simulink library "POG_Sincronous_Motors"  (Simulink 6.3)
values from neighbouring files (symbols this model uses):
  al = Tipo(2)    [Flusso_Rotorico_An.m]
  bm = 0.8*N*metri*secondo/rad    (= 0.8)    [architetture_epicicloidale.m]    (also in architetture_epicicloidale_cont.m; architetture_epicicloidale_HEV.m; architetture_epicicloidale_prova.m; architetture_HEV_controllo.m)
  Iw0 = 0*wI0    [architetture_epicicloidale.m]    (also in architetture_epicicloidale_cont.m = wI0; architetture_epicicloidale_HEV.m; architetture_epicicloidale_prova.m; architetture_HEV_controllo.m)
  Jm = 1.6*kg*metri^2    (= 1.6)    [architetture_epicicloidale.m]    (also in architetture_epicicloidale_cont.m; architetture_epicicloidale_HEV.m = 1.64945909552; architetture_epicicloidale_prova.m; architetture_HEV_controllo.m = 0.529459095518)
  m = 5    [architetture_epicicloidale.m]    (also in architetture_epicicloidale_cont.m; architetture_epicicloidale_HEV.m; architetture_epicicloidale_prova.m; architetture_HEV_controllo.m)
  Nar = 200    [architetture_epicicloidale.m]    (also in architetture_epicicloidale_cont.m; architetture_epicicloidale_HEV.m; architetture_epicicloidale_prova.m; architetture_HEV_controllo.m)
  Nc = 30    [architetture_epicicloidale.m]    (also in architetture_epicicloidale_cont.m; architetture_epicicloidale_HEV.m; architetture_epicicloidale_prova.m; architetture_HEV_controllo.m)
  p = 1    [architetture_epicicloidale.m]    (also in architetture_epicicloidale_cont.m; architetture_epicicloidale_HEV.m; architetture_epicicloidale_prova.m; architetture_HEV_controllo.m)
  Phir = 0.02*Weber    (= 0.02)    [architetture_epicicloidale.m]    (also in architetture_epicicloidale_cont.m; architetture_epicicloidale_HEV.m; architetture_epicicloidale_prova.m; architetture_HEV_controllo.m)
  Star = Si    [architetture_epicicloidale.m]    (also in architetture_epicicloidale_cont.m; architetture_epicicloidale_HEV.m; architetture_epicicloidale_prova.m; architetture_HEV_controllo.m)
  Thm0 = 0    [architetture_epicicloidale.m]    (also in architetture_epicicloidale_cont.m; architetture_epicicloidale_HEV.m; architetture_epicicloidale_prova.m; architetture_HEV_controllo.m)
  Tipo = eval(Flusso(ij).Tipo)    [architetture_epicicloidale.m]    (also in architetture_epicicloidale_cont.m; architetture_epicicloidale_HEV.m; architetture_epicicloidale_prova.m; architetture_HEV_controllo.m)
  Wm0 = 0*Wr_d    (= 0)    [architetture_epicicloidale.m]    (also in architetture_epicicloidale_cont.m = 62.5; architetture_epicicloidale_HEV.m; architetture_epicicloidale_prova.m; architetture_HEV_controllo.m)
undefined symbols (not defined in the file or in its folder): Ls, Ms0, Rs
libraries: simulink x2

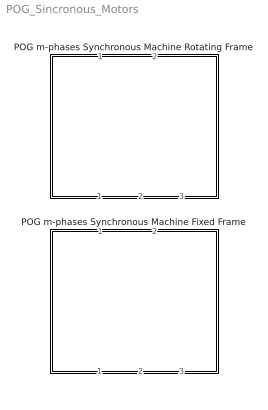
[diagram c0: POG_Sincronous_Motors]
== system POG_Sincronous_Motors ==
  POG m-phases Synchronous Machine Fixed Frame : Subsystem  Orientation=down  mask(POG Multi-Phase Motor (Fixed Frame)){Motor_Par=[m p], Phase_Par=[Nc Star], Electric_Par=[Rs Ls Ms0], Mech_Par=[Jm bm], Plux_Par=[Phir Nar], Iniz_Cond=[Wm0; Thm0; Iw0], TipoFlux=User defined, Tipo=Tipo, alfa=al, degree=6, TipoF=Tipo}
      mask prompts: Motor_Par "Number of phases, Number of polar couples: [m, p] -> [Nr, Nr]"; Phase_Par "Number of coils, Star connected?: [Nc, Star] -> [Nr, (True, False)]"; Electric_Par "Electric Parameters: [Rs, Ls, Ms0] -> [Henry, Henry, Ohm]"; Mech_Par "Mechanical Parameters: [Jm, bm] -> [kg*m^2, N m s/rad]"; Plux_Par "Maximum value of the rotor flux, Number of Fourier harmonics: [Phir, Nar] -> [W, Nr]"; Iniz_Cond "Initial conditions: [Wm0, Thm0, It0] -> [rad/s, rad, A]"; TipoFlux "Type of Rotor Flux"; Tipo "Type defined by user: Tipo -> [Nr,alfa,degree]"; alfa "Flux function parameter: alfa -> [0, pi/2]:"; degree "Degree of the polinomial flux function:"; TipoF "Components of the Fourier series: [9, Nmax, CompAi] -> [9, Nr, a0, a1, ..., aNr]"
      mask help: Multi-Phase Permanent Magnet Synchronous Motor: [m, p] = Number of motor phases, Polar couples; [Nc, Star] = Number of coils per phase, Type of phase connection; [Rs, Ls, Ms0] = Resistance, Self inductance, Mutual inductance of each phase; [Jm, bm] = Inertia momentum, Friction coefficient of the rotor; [Phir, Nar] = Maximum value of the rotor flux, Number of Fourier harmonics; [Wm0, Thm0, Iw0] = Initial conditions on Velocity, Position of the motor and Currents; Type of Rotor Flux (Tipo): Trapezoidal [1,alfa]; Triangular [1, 0]; Squared wave [2]; Sinusoidal [3]; Cosinusoidally connected [4,alf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
      mask init:
      | m=Motor_Par(1);
      | p=Motor_Par(2);
      | Nc=Phase_Par(1);
      | Star=Phase_Par(2);
      | Rs=Electric_Par(1);
      | Ls=Electric_Par(2);
      | Ms0=Electric_Par(3);
      | Jm=Mech_Par(1);
      | bm=Mech_Par(2);
      | Phir=Plux_Par(1);
      | Nar=Plux_Par(2);
      | 
      | %%%%%%%%%%%%%%%%%%%%% Initial Conditions
      | if length(Iniz_Cond)<(m+2-Star)
      |     Iniz_Cond=[Iniz_Cond 0*[1:m+2-Star-length(Iniz_Cond)]];
      |     disp('Correction: Iniz_Cond = ...');
      |     disp(Iniz_Cond)
      | end
      | Wm0 = Iniz_Cond(1);
      | Thm0= Iniz_Cond(2);
      | Ibt0 = Iniz_Cond(3:m+2-Star);
      | 
      | %%%%%%%%%%%%%%%%%%%%%%%%%%%%
      | FluxName(1)=struct('Nome','Trapezoidal');
      | FluxName(2)=struct('Nome','Squared wave');
      | FluxName(3)=struct('Nome','Sinusoidal');
      | FluxName(4)=struct('Nome','Cosinusoidally connected');
      | FluxName(5)=struct('Nome','Sinusoidally connected');
      | FluxName(6)=struct('Nome','Polynomial even');
      | FluxName(7)=struct('Nome','Polynomial odd');
      | FluxName(8)=struct('Nome','Trapezoidal if derived');
      | FluxName(9)=struct('Nome','Fourier defined');
      | 
      | switch TipoFlux
      |     case 'User defined',
      |     case 'Trapezoidal'
      |         if alfa<0, alfa=0; disp('Correction: alfa = 0'); end
      |         if alfa>pi/2, alfa=pi/2; disp('Correction: alfa = pi/2'); end
      |         Tipo = [1,alfa];
      |     case 'Triangular'
      |         Tipo = [1,  0];
      |     case 'Squared wave'
      |         Tipo = [2];
      |     case 'Sinusoidal'
      |         Tipo = [3];
      |     case 'Cosinusoidally connected'
      |         if alfa<0, alfa=0; disp('Correction: alfa = 0'); end
      |         if alfa>pi/2, alfa=pi/2; disp('Correction: alfa = pi/2'); end
      |         Tipo = [4,alfa];
      |     case 'Sinusoidally connected'
      |         if alfa<0, alfa=0; disp('Correction: alfa = 0'); end
      |         if alfa>pi/2, alfa=pi/2; disp('Correction: alfa = pi/2'); end
      |         Tipo = [5,alfa];
      |     case 'Polynomial even'
      |         if alfa<0, alfa=0; disp('Correction: alfa = 0'); end
      |         if alfa>pi/2, alfa=pi/2; disp('Correction: alfa = pi/2'); end
      |         if rem(degree)==1, 
      |             degree=degree-1; 
      |             disp(['Correction: degree = ' num2str(degree)]); 
      |         end
      |         if degree<2
      |             degree=2; 
      |             disp(['Correction: degree = ' num2str(degree)]); 
      |         end            
      |         Tipo = [6,alfa,degree];
      |     case 'Polynomial odd'
      |         if alfa<0, alfa=0; disp('Correction: alfa = 0'); end
      |         if alfa>pi/2, alfa=pi/2; disp('Correction: alfa = pi/2'); end
      |         if rem(degree)==0, 
      |             degree=degree-1; 
      |             disp(['Correction: degree = ' num2str(degree)]); 
      |         end
      |         if degree<1
      |             degree=1; 
      |             disp(['Correction: degree = ' num2str(degree)]); 
      |         end            
      |         Tipo = [7,alfa,degree];
      |     case 'Trapezoidal if derived'
      |         Tipo = [8,alfa];
      |         if alfa<0, alfa=0; disp('Correction: alfa = 0'); end
      |         if alfa>pi/2, alfa=pi/2; disp('Correction: alfa = pi/2'); end
      |     case 'Fourier defined'
      |         if TipoF(1)~=9
      |             disp('Correction: NrType = 9 (Fourier defined)')
      |             TipoF(1)=9;
      |         end
      |         if length(TipoF)<2
      |             TipoF(2)=m;
      |             disp('Correction: Fourier defined -> TipoF = ...');
      |             disp(TipoF)
      |         end
      |         if TipoF(2)<m,
      |             TipoF(2)=m;
      |             disp('Correction: Fourier defined -> Nas = m');
      |         end
      |         if length(TipoF)<(TipoF(2)+3)
      |             TipoF=[TipoF 0*[1:TipoF(2)+3-length(TipoF)]];
      |             disp('Correction: Fourier defined -> TipoF = ...'); 
      |             disp(TipoF)
      |         end
      |         Tipo = TipoF;   % [9,Nmax,CompAi]
      |     otherwise,
      |         disp('Flux type not correct')
      |         return
      | end
      | 
      | switch TipoFlux
      |     case 'User defined',
      |         disp(['The rotor flux is ''''' FluxName(Tipo(1)).Nome ''''' (Us. Def.)'])
      |     otherwise,
      |         disp(['The rotor flux is ''''' TipoFlux ''''''])
      | end
      | 
      | %%%%%% Trasformazione "T(b->t)"
      | %%%%%% matrice tTb=T_b_Concordia_Sincrono(m); 
      | if rem(m,2)==0
      |     disp(['Warning (T_b_Concordia_Sincrono): m = ' num2str(m) ' è pari']) 
      | end
      | tTb = ones(m)/sqrt(2);
      | w = 2*pi/m;
      | for k = [1:2:m-2]
      |     for h = [0:m-1]
      |         tTb(h+1,k  ) = cos(h*k*w);
      |         tTb(h+1,k+1) = sin(h*k*w);
      |     end
      | end
      | tTb=sqrt(2/m)*tTb;
      | 
      | %%%%%% Auto and mutual inductance matrix  wLs(MLb) defined in the rotating frame
      | Ls0 = Ls-Ms0;
      | MLb = p*eye(m)*Ls0;         
      | MLb(1,1)=p*(Ls0+m*Ms0/2);  
      | MLb(2,2)=p*(Ls0+m*Ms0/2);
      | 
      | %%%%%% Resistance matrice wRs(MR) defined in the rotating frame
      | MR = p*Rs*eye(m);   
      | 
      | %%%%%% Calcolo del vetore di coppia Ktau
      | Phic = p*Nc*Phir;   %%% Maximum concatenated flux;
      | if Nar<m,           %%% Nar = numero di compenenti spettrali dello svilupo in serie
      |     Nar=m;  disp('Correction: Nar = m');
      | end
      | 
      | %%%%%% Reduction of the system matrices if Star is True
      | if Star                     
      |     tTabc=tTb(:,[1:m-1]);
      |     MLabc=MLb([1:m-1],[1:m-1]);
      |     MRabc=MR([1:m-1],[1:m-1]);
      |     Ibt0=MLabc*Ibt0;
      | else
      |     tTabc=eye(m);
      |     MLabc=tTb*MLb*tTb';
      |     MRabc=tTb*MR*tTb';
      |     Ibt0=MLabc*tTabc'*Ibt0;
      | end
      | Sfasa  = -2*pi*[0:m-1]'/m;   % Matrice di sfasamento
      | LkUpT_in=[-1:0.0001:1]*2*pi;
      | LkUpT_out=0*LkUpT_in;
      | for n=[1:2:Nar]
      |     LkUpT_out=LkUpT_out-Flusso_Rotorico_An(Tipo,n)*n*sin(n*LkUpT_in);
      | end
      | LkUpT_out=p*Phic*LkUpT_out;
  POG m-phases Synchronous Machine Rotating Frame : Subsystem  Orientation=down  mask(POG Multi-Phase Motor (Rotating Frame)){Motor_Par=[m p], Phase_Par=[Nc Star], Electric_Par=[Rs Ls Ms0], Mech_Par=[Jm bm], Plux_Par=[Phir Nar], Iniz_Cond=[Wm0; Thm0; Iw0], TipoFlux=User defined, Tipo=Tipo, alfa=al, degree=6, TipoF=Tipo}
      mask prompts: Motor_Par "Number of phases, Number of polar couples: [m, p] -> [Nr, Nr]"; Phase_Par "Number of coils, Star connected?: [Nc, Star] -> [Nr, (True, False)]"; Electric_Par "Electric Parameters: [Rs, Ls, Ms0] -> [Henry, Henry, Ohm]"; Mech_Par "Mechanical Parameters: [Jm, bm] -> [kg*m^2, N m s/rad]"; Plux_Par "Maximum value of the rotor flux, Number of Fourier harmonics: [Phir, Nar] -> [W, Nr]"; Iniz_Cond "Initial conditions: [Wm0, Thm0, Iw0] -> [rad/s, rad, A]"; TipoFlux "Type of Rotor Flux"; Tipo "Type defined by user: Tipo -> [Nr,alfa,degree]"; alfa "Flux function parameter: alfa -> [0, pi/2]:"; degree "Degree of the polinomial flux function:"; TipoF "Components of the Fourier series: [9, Nmax, CompAi] -> [9, Nr, a0, a1, ..., aNr]"
      mask help: Multi-Phase Permanent Magnet Synchronous Motor: [m, p] = Number of motor phases, Polar couples; [Nc, Star] = Number of coils per phase, Type of phase connection; [Rs, Ls, Ms0] = Resistance, Self inductance, Mutual inductance of each phase; [Jm, bm] = Inertia momentum, Friction coefficient of the rotor; [Phir, Nar] = Maximum value of the rotor flux, Number of Fourier harmonics; [Wm0, Thm0, Iw0] = Initial conditions on Velocity, Position of the motor and Currents; Type of Rotor Flux (Tipo): Trapezoidal [1,alfa]; Triangular [1, 0]; Squared wave [2]; Sinusoidal [3]; Cosinusoidally connected [4,alf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
      mask init:
      | m=Motor_Par(1);
      | p=Motor_Par(2);
      | Nc=Phase_Par(1);
      | Star=Phase_Par(2);
      | Rs=Electric_Par(1);
      | Ls=Electric_Par(2);
      | Ms0=Electric_Par(3);
      | Jm=Mech_Par(1);
      | bm=Mech_Par(2);
      | Phir=Plux_Par(1);
      | Nar=Plux_Par(2);
      | 
      | %%%%%%%%%%%%%%%%%%%%% Initial Conditions
      | if length(Iniz_Cond)<(m+2-Star)
      |     Iniz_Cond=[Iniz_Cond 0*[1:m+2-Star-length(Iniz_Cond)]];
      |     disp('Correction: Iniz_Cond = ...');
      |     disp(Iniz_Cond)
      | end
      | Wm0 = Iniz_Cond(1);
      | Thm0= Iniz_Cond(2);
      | Iw0 = Iniz_Cond(3:m+2-Star);
      | 
      | %%%%%%%%%%%%%%%%%%%%%%%%%%%%
      | FluxName(1)=struct('Nome','Trapezoidal');
      | FluxName(2)=struct('Nome','Squared wave');
      | FluxName(3)=struct('Nome','Sinusoidal');
      | FluxName(4)=struct('Nome','Cosinusoidally connected');
      | FluxName(5)=struct('Nome','Sinusoidally connected');
      | FluxName(6)=struct('Nome','Polynomial even');
      | FluxName(7)=struct('Nome','Polynomial odd');
      | FluxName(8)=struct('Nome','Trapezoidal if derived');
      | FluxName(9)=struct('Nome','Fourier defined');
      | 
      | switch TipoFlux
      |     case 'User defined',
      |     case 'Trapezoidal'
      |         if alfa<0, alfa=0; disp('Correction: alfa = 0'); end
      |         if alfa>pi/2, alfa=pi/2; disp('Correction: alfa = pi/2'); end
      |         Tipo = [1,alfa];
      |     case 'Triangular'
      |         Tipo = [1,  0];
      |     case 'Squared wave'
      |         Tipo = [2];
      |     case 'Sinusoidal'
      |         Tipo = [3];
      |     case 'Cosinusoidally connected'
      |         if alfa<0, alfa=0; disp('Correction: alfa = 0'); end
      |         if alfa>pi/2, alfa=pi/2; disp('Correction: alfa = pi/2'); end
      |         Tipo = [4,alfa];
      |     case 'Sinusoidally connected'
      |         if alfa<0, alfa=0; disp('Correction: alfa = 0'); end
      |         if alfa>pi/2, alfa=pi/2; disp('Correction: alfa = pi/2'); end
      |         Tipo = [5,alfa];
      |     case 'Polynomial even'
      |         if alfa<0, alfa=0; disp('Correction: alfa = 0'); end
      |         if alfa>pi/2, alfa=pi/2; disp('Correction: alfa = pi/2'); end
      |         if rem(degree)==1, 
      |             degree=degree-1; 
      |             disp(['Correction: degree = ' num2str(degree)]); 
      |         end
      |         if degree<2
      |             degree=2; 
      |             disp(['Correction: degree = ' num2str(degree)]); 
      |         end            
      |         Tipo = [6,alfa,degree];
      |     case 'Polynomial odd'
      |         if alfa<0, alfa=0; disp('Correction: alfa = 0'); end
      |         if alfa>pi/2, alfa=pi/2; disp('Correction: alfa = pi/2'); end
      |         if rem(degree)==0, 
      |             degree=degree-1; 
      |             disp(['Correction: degree = ' num2str(degree)]); 
      |         end
      |         if degree<1
      |             degree=1; 
      |             disp(['Correction: degree = ' num2str(degree)]); 
      |         end            
      |         Tipo = [7,alfa,degree];
      |     case 'Trapezoidal if derived'
      |         Tipo = [8,alfa];
      |         if alfa<0, alfa=0; disp('Correction: alfa = 0'); end
      |         if alfa>pi/2, alfa=pi/2; disp('Correction: alfa = pi/2'); end
      |     case 'Fourier defined'
      |         if TipoF(1)~=9
      |             disp('Correction: NrType = 9 (Fourier defined)')
      |             TipoF(1)=9;
      |         end
      |         if length(TipoF)<2
      |             TipoF(2)=m;
      |             disp('Correction: Fourier defined -> TipoF = ...');
      |             disp(TipoF)
      |         end
      |         if TipoF(2)<m,
      |             TipoF(2)=m;
      |             disp('Correction: Fourier defined -> Nas = m');
      |         end
      |         if length(TipoF)<(TipoF(2)+3)
      |             TipoF=[TipoF 0*[1:TipoF(2)+3-length(TipoF)]];
      |             disp('Correction: Fourier defined -> TipoF = ...'); 
      |             disp(TipoF)
      |         end
      |         Tipo = TipoF;   % [9,Nmax,CompAi]
      |     otherwise,
      |         disp('Flux type not correct')
      |         return
      | end
      | 
      | switch TipoFlux
      |     case 'User defined',
      |         disp(['The rotor flux is ''''' FluxName(Tipo(1)).Nome ''''' (Us. Def.)'])
      |     otherwise,
      |         disp(['The rotor flux is ''''' TipoFlux ''''''])
      | end
      | 
      | 
      | %%%%%% Trasformazione "T(b->t)"
      | %%%%%% matrice tTb=T_b_Concordia_Sincrono(m); 
      | if rem(m,2)==0
      |     disp(['Warning (T_b_Concordia_Sincrono): m = ' num2str(m) ' è pari']) 
      | end
      | tTb = ones(m)/sqrt(2);
      | w = 2*pi/m;
      | for k = [1:2:m-2]
      |     for h = [0:m-1]
      |         tTb(h+1,k  ) = cos(h*k*w);
      |         tTb(h+1,k+1) = sin(h*k*w);
      |     end
      | end
      | tTb=sqrt(2/m)*tTb;    
      | 
      | %%%%%% Trasformazione "T(b->w)": matrici I_m, MKr e Jr;
      | I_m = eye(m);
      | MKr = zeros(m);              
      | Jr  = zeros(m);
      | for k=[1:2:m-1]
      |     MKr(k,k ) = k;  MKr(k+1,k+1) = k;
      |     Jr(k+1,k) = 1;  Jr(k,k+1) = -1;  
      | end
      | 
      | %%%%%% Auto and mutual inductance matrix  wLs(MLb) defined in the rotating frame
      | Ls0 = Ls-Ms0;
      | MLb = p*eye(m)*Ls0;         
      | MLb(1,1)=p*(Ls0+m*Ms0/2);  
      | MLb(2,2)=p*(Ls0+m*Ms0/2);
      | 
      | %%%%%% Resistance matrice wRs(MR) defined in the rotating frame
      | MR = p*Rs*eye(m);           
      | 
      | %%%%%% Vector Kr for the energy redistribution wJs*wJs ("j*w*L")
      | Kr= zeros(m,1);             
      | for k=[1:2:m-1]
      |     Kr(k)= k;  Kr(k+1)= k;
      | end
      | 
      | %%%%%% Calcolo del vetore di coppia Ktau
      | Phic = p*Nc*Phir;   %%% Maximum concatenated flux;
      | if Nar<m,           %%% Nar = numero di compenenti spettrali dello svilupo in serie
      |     Nar=m;  disp('Correction: Nar = m');
      | end
      | N_2m_2m=[0:2*m:Nar]';  %%% Matrices N_2m_2m, N_m_2m, An_sin, An_sin, M_gira
      | N_m_2m =[m:2*m:Nar]'; 
      | An_sin=zeros((m-1)/2,max(size(N_2m_2m)));
      | An_cos=zeros((m-1)/2,max(size(N_2m_2m)));
      | for k=[1:2:m-1]
      |     An_piu_k = Flusso_Rotorico_An(Tipo,N_2m_2m+k)';
      |     An_men_k = Flusso_Rotorico_An(Tipo,N_2m_2m-k)';
      |     An_sin((k+1)/2,:) = -p*sqrt(m/2)*Phic*(An_piu_k.*(N_2m_2m'+k) + An_men_k.*(N_2m_2m'-k));
      |     An_cos((k+1)/2,:) =  p*sqrt(m/2)*Phic*(An_piu_k.*(N_2m_2m'+k) - An_men_k.*(N_2m_2m'-k));
      | end
      | An_m_sin = -p*sqrt(m)*Phic*(Flusso_Rotorico_An(Tipo,N_m_2m)').*N_m_2m';
      | M_gira=eye(m);
      | M_gira=[M_gira(:,1:2:m-1) M_gira(:,2:2:m-1) M_gira(:,m)];
      | %
      | if Star        %%% Reduction of the system matrices if Star is True
      |     tTb=tTb(:,[1:m-1]);
      |     MKr=MKr([1:m-1],[1:m-1]);
      |     Jr=Jr([1:m-1],[1:m-1]);
      |     I_m=eye(m-1);
      |     MLb=MLb([1:m-1],[1:m-1]);
      |     MR=MR([1:m-1],[1:m-1]);
      |     Kr=Kr([1:m-1]);
      |     M_gira=M_gira([1:m-1],:);
      | end
      | %

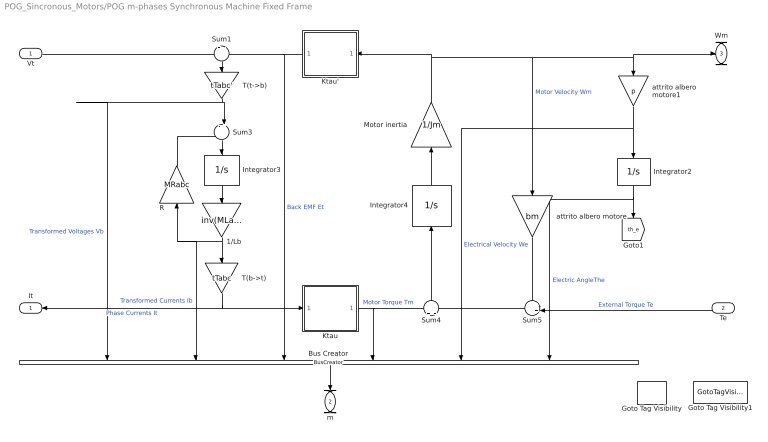
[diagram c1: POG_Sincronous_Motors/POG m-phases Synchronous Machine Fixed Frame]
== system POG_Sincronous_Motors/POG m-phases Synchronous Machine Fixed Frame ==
  Vt : Inport
  Te : Inport  Orientation=left  Port=2
  1/Lb : Gain  Orientation=down  Gain=inv(MLabc)  Multiplication=Matrix(K*u) (u vector)
  Bus Creator : BusCreator  Orientation=down  Inputs=6
  Goto Tag Visibility : GotoTagVisibility
  Goto Tag Visibility1 : GotoTagVisibility
  Integrator2 : Integrator  Orientation=down  InitialCondition=Thm0*p
  Integrator3 : Integrator  Orientation=down  InitialCondition=Ibt0
  Integrator4 : Integrator  Orientation=up  InitialCondition=Wm0*Jm
  Ktau : Subsystem
  Ktau' : Subsystem  Orientation=left
  Motor inertia : Gain  Orientation=up  Gain=1/Jm
  R : Gain  Orientation=up  Gain=MRabc  Multiplication=Matrix(K*u) (u vector)
  Sum1 : Sum  Orientation=down  Inputs=+|-
  Sum3 : Sum  Orientation=down  Inputs=-+|
  Sum4 : Sum  Orientation=up  Inputs=+|-
  Sum5 : Sum  Orientation=left  Inputs=++|
  T(b->t) : Gain  Orientation=down  Gain=tTabc  Multiplication=Matrix(K*u) (u vector)
  T(t->b) : Gain  Orientation=down  Gain=tTabc'  Multiplication=Matrix(K*u) (u vector)
  attrito albero motore : Gain  Orientation=down  Gain=bm
  attrito albero motore1 : Gain  Orientation=down  Gain=p
  It : Outport  Orientation=left
  m : Outport  Orientation=down  Port=2
  Wm : Outport  Port=3
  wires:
  Sum5/1 -> Sum4/2
  attrito albero motore1/1 -> Integrator2/1, Bus Creator/5  "Electrical Velocity We"
  Integrator2/1 -> [th_e], Bus Creator/6  "Electric AngleThe"
  Ktau/1(Tm) -> Sum4/1, Bus Creator/4  "Motor Torque Tm"
  Sum4/1 -> Integrator4/1
  Integrator4/1 -> Motor inertia/1
  Motor inertia/1 -> Ktau'/1(Wm), attrito albero motore/1, attrito albero motore1/1, Wm/1  "Motor Velocity Wm"
  attrito albero motore/1 -> Sum5/1
  Te/1 -> Sum5/2  "External Torque Te"
  Bus Creator/1 -> m/1
  Integrator3/1 -> 1/Lb/1
  1/Lb/1 -> T(b->t)/1, R/1, Bus Creator/2  "Transformed Currents Ib"
  Sum3/1 -> Integrator3/1
  Sum1/1 -> T(t->b)/1
  Vt/1 -> Sum1/1
  T(b->t)/1 -> It/1, Ktau/1(It)  "Phase Currents It"
  Ktau'/1(Et) -> Sum1/2, Bus Creator/3  "Back EMF Et"
  R/1 -> Sum3/1
  T(t->b)/1 -> Sum3/2, Bus Creator/1  "Transformed Voltages Vb"

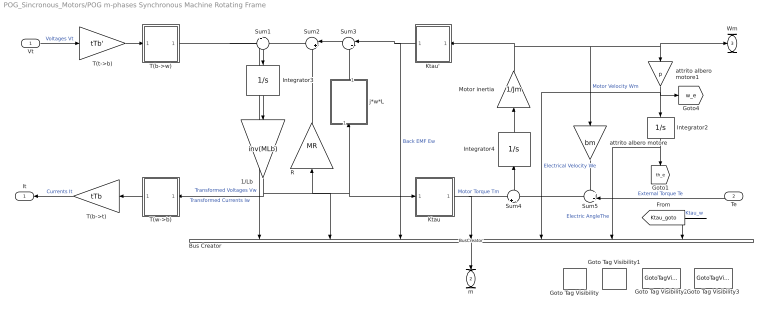
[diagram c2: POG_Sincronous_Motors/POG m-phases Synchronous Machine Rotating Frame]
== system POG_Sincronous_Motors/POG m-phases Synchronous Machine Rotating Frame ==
  Vt : Inport
  Te : Inport  Orientation=left  Port=2
  1/Lb : Gain  Orientation=down  Gain=inv(MLb)  Multiplication=Matrix(K*u) (u vector)
  Bus Creator : BusCreator  Orientation=down  Inputs=7
  Goto Tag Visibility{,1..3} (4 alike) : GotoTagVisibility
  Integrator2 : Integrator  Orientation=down  InitialCondition=Thm0*p
  Integrator3 : Integrator  Orientation=down  InitialCondition=MLb*Iw0
  Integrator4 : Integrator  Orientation=up  InitialCondition=Wm0*Jm
  Ktau : Subsystem
  Ktau' : Subsystem  Orientation=left
  Motor inertia : Gain  Orientation=up  Gain=1/Jm
  R : Gain  Orientation=up  Gain=MR  Multiplication=Matrix(K*u) (u vector)
  Sum1 : Sum  Orientation=down  Inputs=+|-
  Sum2 : Sum  Orientation=left  Inputs=|++
  Sum3 : Sum  Orientation=left  Inputs=|++
  Sum4 : Sum  Orientation=up  Inputs=+|-
  Sum5 : Sum  Orientation=left  Inputs=++|
  T(b->t) : Gain  Orientation=left  Gain=tTb  Multiplication=Matrix(K*u) (u vector)
  T(b->w) : Subsystem
  T(t->b) : Gain  Gain=tTb'  Multiplication=Matrix(K*u) (u vector)
  T(w->b) : Subsystem  Orientation=left
  attrito albero motore : Gain  Orientation=down  Gain=bm
  attrito albero motore1 : Gain  Orientation=down  Gain=p
  j*w*L : Subsystem  Orientation=up
  It : Outport  Orientation=left
  m : Outport  Orientation=down  Port=2
  Wm : Outport  Port=3
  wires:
  Bus Creator/1 -> m/1
  T(b->t)/1 -> It/1  "Currents It"
  Te/1 -> Sum5/2  "External Torque Te"
  Vt/1 -> T(t->b)/1  "Voltages Vt"
  T(w->b)/1(It) -> T(b->t)/1
  T(b->w)/1(Vw) -> Bus Creator/1, Sum1/1  "Transformed Voltages Vw"
  attrito albero motore/1 -> Sum5/1
  Motor inertia/1 -> Ktau'/1(Wm), Wm/1, attrito albero motore1/1, attrito albero motore/1  "Motor Velocity Wm"
  Integrator4/1 -> Motor inertia/1
  Sum4/1 -> Integrator4/1
  Ktau'/1(Ew) -> Bus Creator/3, Sum3/1  "Back EMF Ew"
  Ktau/1(Tm) -> Bus Creator/4, Sum4/1  "Motor Torque Tm"
  j*w*L/1(Out1) -> Sum3/2
  Sum3/1 -> Sum2/1
  R/1 -> Sum2/2
  Sum2/1 -> Sum1/2
  1/Lb/1 -> Bus Creator/2, Ktau/1(Iw), j*w*L/1(In1), R/1, T(w->b)/1(Iw)  "Transformed Currents Iw"
  Integrator3/1 -> 1/Lb/1
  Sum1/1 -> Integrator3/1
  Integrator2/1 -> Bus Creator/6, [th_e]  "Electric AngleThe"
  attrito albero motore1/1 -> [w_e], Integrator2/1, Bus Creator/5  "Electrical Velocity We"
  T(t->b)/1 -> T(b->w)/1(Vt)
  Sum5/1 -> Sum4/2
  [Ktau_goto] -> Bus Creator/7  "Ktau_w"

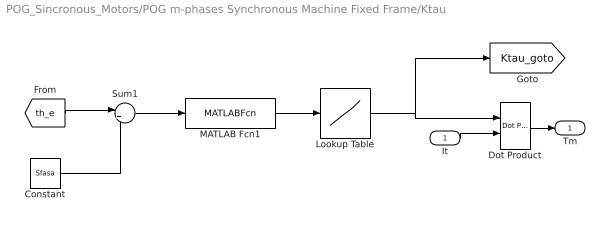
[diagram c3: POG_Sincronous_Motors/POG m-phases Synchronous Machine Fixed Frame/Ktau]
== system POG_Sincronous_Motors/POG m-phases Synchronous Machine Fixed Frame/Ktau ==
  It : Inport
  Constant : Constant  Value=Sfasa  VectorParams1D=off
  Dot Product : simulink/Math Operations/Dot Product  InputSameDT=on  OutDataType=sfix(16)  OutScaling=2^-10  DoSatur=off
  Lookup Table : Lookup  InputValues=LkUpT_in  OutputValues=LkUpT_out
  MATLAB Fcn1 : MATLABFcn  MATLABFcn=rem(u,2*pi)
  Sum1 : Sum  Inputs=|++
  Tm : Outport
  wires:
  Dot Product/1 -> Tm/1
  It/1 -> Dot Product/2
  Lookup Table/1 -> Dot Product/1, [Ktau_goto]
  MATLAB Fcn1/1 -> Lookup Table/1
  [th_e] -> Sum1/1
  Sum1/1 -> MATLAB Fcn1/1
  Constant/1 -> Sum1/2

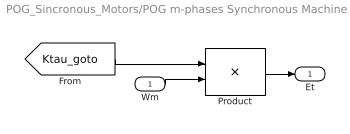
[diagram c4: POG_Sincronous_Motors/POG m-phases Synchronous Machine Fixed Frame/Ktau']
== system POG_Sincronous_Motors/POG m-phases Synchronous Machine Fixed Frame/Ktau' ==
  Wm : Inport
  Product : Product  Multiplication=Matrix(*)
  Et : Outport
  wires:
  Wm/1 -> Product/2
  Product/1 -> Et/1
  [Ktau_goto] -> Product/1

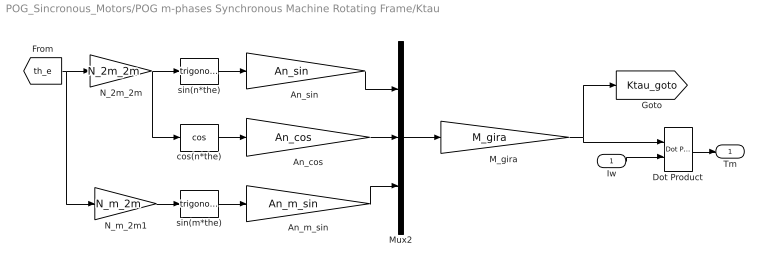
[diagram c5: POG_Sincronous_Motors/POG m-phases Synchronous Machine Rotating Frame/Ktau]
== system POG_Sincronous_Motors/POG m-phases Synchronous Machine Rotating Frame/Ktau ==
  Iw : Inport
  An_cos : Gain  Gain=An_cos  Multiplication=Matrix(K*u) (u vector)
  An_m_sin : Gain  Gain=An_m_sin  Multiplication=Matrix(K*u) (u vector)
  "An_sin " : Gain  Gain=An_sin  Multiplication=Matrix(K*u) (u vector)
  Dot Product : simulink/Math Operations/Dot Product  InputSameDT=on  OutDataType=sfix(16)  OutScaling=2^-10  DoSatur=off
  "M_gira " : Gain  Gain=M_gira  Multiplication=Matrix(K*u) (u vector)
  Mux2 : Mux  Inputs=3
  N_2m_2m : Gain  Gain=N_2m_2m  Multiplication=Matrix(K*u) (u vector)
  N_m_2m1 : Gain  Gain=N_m_2m  Multiplication=Matrix(K*u) (u vector)
  cos(n*the) : Trigonometry  Operator=cos
  sin(m*the) : Trigonometry
  sin(n*the) : Trigonometry
  Tm : Outport
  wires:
  An_m_sin/1 -> Mux2/3
  "M_gira "/1 -> [Ktau_goto], Dot Product/1
  Mux2/1 -> "M_gira "/1
  An_cos/1 -> Mux2/2
  "An_sin "/1 -> Mux2/1
  sin(m*the)/1 -> An_m_sin/1
  N_m_2m1/1 -> sin(m*the)/1
  cos(n*the)/1 -> An_cos/1
  sin(n*the)/1 -> "An_sin "/1
  N_2m_2m/1 -> cos(n*the)/1, sin(n*the)/1
  [th_e] -> N_m_2m1/1, N_2m_2m/1
  Iw/1 -> Dot Product/2
  Dot Product/1 -> Tm/1

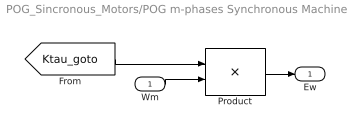
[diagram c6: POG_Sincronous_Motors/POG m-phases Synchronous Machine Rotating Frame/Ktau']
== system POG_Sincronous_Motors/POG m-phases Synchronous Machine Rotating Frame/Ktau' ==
  Wm : Inport
  Product : Product  Multiplication=Matrix(*)
  Ew : Outport
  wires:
  [Ktau_goto] -> Product/1
  Product/1 -> Ew/1
  Wm/1 -> Product/2

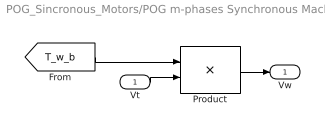
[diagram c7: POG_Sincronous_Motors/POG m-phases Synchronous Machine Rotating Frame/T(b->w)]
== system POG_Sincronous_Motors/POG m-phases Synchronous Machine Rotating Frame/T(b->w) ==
  Vt : Inport
  Product : Product  Multiplication=Matrix(*)
  Vw : Outport
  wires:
  [T_w_b] -> Product/1
  Product/1 -> Vw/1
  Vt/1 -> Product/2

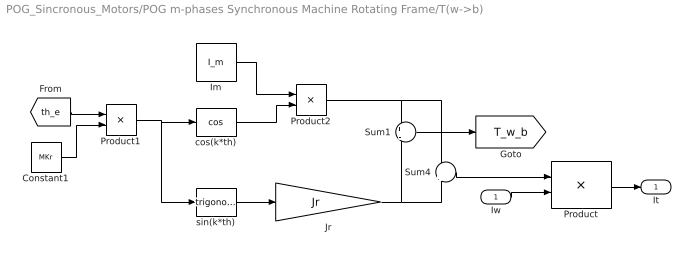
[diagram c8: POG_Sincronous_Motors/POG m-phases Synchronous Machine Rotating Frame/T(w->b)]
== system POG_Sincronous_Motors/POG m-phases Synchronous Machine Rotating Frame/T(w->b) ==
  Iw : Inport
  Constant1 : Constant  Value=MKr
  Im : Constant  Value=I_m  VectorParams1D=off
  Jr : Gain  Gain=Jr  Multiplication=Matrix(K*u)
  Product : Product  Multiplication=Matrix(*)
  Product1 : Product
  Product2 : Product
  Sum1 : Sum  Inputs=+|-
  Sum4 : Sum  Inputs=+|+
  cos(k*th) : Trigonometry  Operator=cos
  sin(k*th) : Trigonometry
  It : Outport
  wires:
  Sum1/1 -> [T_w_b]
  sin(k*th)/1 -> Jr/1
  [th_e] -> Product1/1
  Constant1/1 -> Product1/2
  Product1/1 -> cos(k*th)/1, sin(k*th)/1
  cos(k*th)/1 -> Product2/2
  Im/1 -> Product2/1
  Product2/1 -> Sum1/1, Sum4/1
  Jr/1 -> Sum1/2, Sum4/2
  Iw/1 -> Product/2
  Product/1 -> It/1
  Sum4/1 -> Product/1

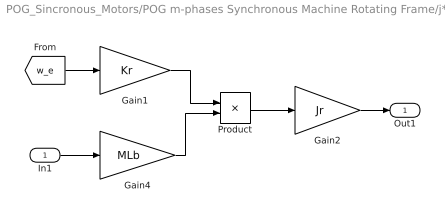
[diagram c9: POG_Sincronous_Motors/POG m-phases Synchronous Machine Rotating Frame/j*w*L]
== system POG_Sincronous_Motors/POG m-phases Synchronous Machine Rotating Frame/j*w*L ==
  In1 : Inport
  Gain1 : Gain  Gain=Kr  Multiplication=Matrix(K*u) (u vector)
  Gain2 : Gain  Gain=Jr  Multiplication=Matrix(K*u) (u vector)
  Gain4 : Gain  Gain=MLb  Multiplication=Matrix(K*u) (u vector)
  Product : Product
  Out1 : Outport
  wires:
  Gain2/1 -> Out1/1
  Product/1 -> Gain2/1
  Gain4/1 -> Product/2
  Gain1/1 -> Product/1
  [w_e] -> Gain1/1
  In1/1 -> Gain4/1
